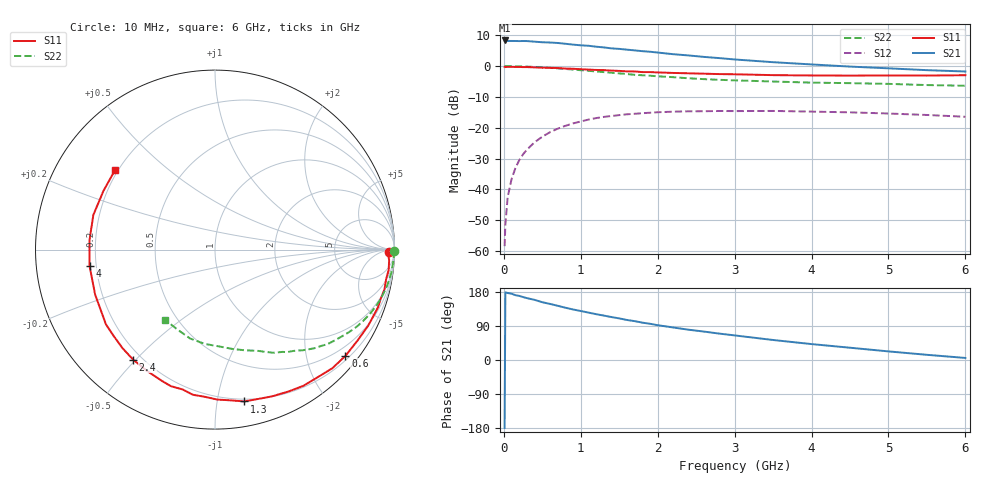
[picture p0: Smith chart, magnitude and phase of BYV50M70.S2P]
! SIEMENS Small Signal Semiconductors
! BFY420
! Si NPN RF SIEGET Grounded Emitter Transistor in MICRO-X
! VCE = 0.5 V  IC = 0.7 mA
! Common Emitter S-Parameters:  October  1996
# GHz  S  MA  R  50
!  f  S11  S21  S12  S22
! GHz  MAG  ANG  MAG  ANG  MAG  ANG  MAG  ANG
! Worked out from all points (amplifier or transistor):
!   36 points, 10 MHz to 6 GHz, reference 50 ohm
!   highest |S21| = 8.3 dB at 10 MHz (marker M1)
!   |S21| within 3 dB of that: start of sweep to 1.608 GHz
!   unconditionally stable (mu >= 1): 4.656 GHz to end of sweep
!   at 250 MHz: K = 0.05, MSG = 18.4 dB, |S12| = -28.6 dB
!   at 1.4 GHz: K = 0.25, MSG = 11.0 dB, |S12| = -16.2 dB
!   at 6 GHz: K = 1.33, MAG = 3.9 dB, |S12| = -16.4 dB
!   S11 on the Smith chart (normalised r, x): 10 MHz: 53, -29; 600 MHz: 0.29, -2.78; 1.3 GHz: 0.18, -1.19; 2.4 GHz: 0.17, -0.49; 4 GHz: 0.17, -0.06; 6 GHz: 0.19, +0.34
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0.01  0.9715 -0.9  2.605 -179.3  0.0012 101.0  0.9982 -0.4
0.02  0.9641 -1.5  2.6 178.7  0.0027 87.7  0.9961 -0.7
0.05  0.972 -3.4  2.556 176.8  0.0075 88.0  0.9967 -1.9
0.1  0.9743 -6.7  2.557 175.0  0.0146 85.5  0.9952 -3.9
0.15  0.9674 -9.9  2.553 171.1  0.0221 82.9  0.9926 -5.8
0.2  0.9699 -13.1  2.544 169.2  0.0298 81.4  0.9911 -7.5
0.3  0.9635 -19.5  2.546 163.3  0.0442 77.3  0.981 -11.5
0.5  0.9419 -32.7  2.436 152.5  0.0716 68.1  0.9545 -18.6
0.6  0.9373 -39.2  2.412 148.0  0.0846 64.0  0.9368 -22.1
0.8  0.9123 -51.3  2.302 138.0  0.1074 55.8  0.8984 -28.6
1.1  0.8772 -68.8  2.137 125.1  0.1356 45.1  0.8378 -37.1
1.3  0.8616 -79.1  2.008 117.2  0.15 38.5  0.799 -42.2
1.6  0.8216 -94.2  1.848 105.6  0.1652 29.8  0.7426 -49.1
1.8  0.7997 -103.1  1.747 98.6  0.1721 24.8  0.7103 -52.8
2.2  0.7744 -119.6  1.56 85.9  0.1823 15.4  0.661 -60.4
2.4  0.764 -126.7  1.489 80.0  0.1846 11.7  0.6345 -63.9
2.8  0.7418 -139.6  1.348 69.7  0.187 4.7  0.5989 -69.9
3.5  0.7133 -159.5  1.157 52.8  0.1873 -4.9  0.5624 -79.9
4  0.7048 -172.7  1.064 42.0  0.1828 -11.0  0.5393 -87.9
4.5  0.7011 175.6  0.982 32.4  0.1777 -16.6  0.5288 -95.9
5.5  0.7025 152.1  0.859 13.7  0.1611 -24.6  0.4924 -115.0
6  0.7116 141.5  0.817 5.4  0.1506 -26.6  0.4798 -125.7
